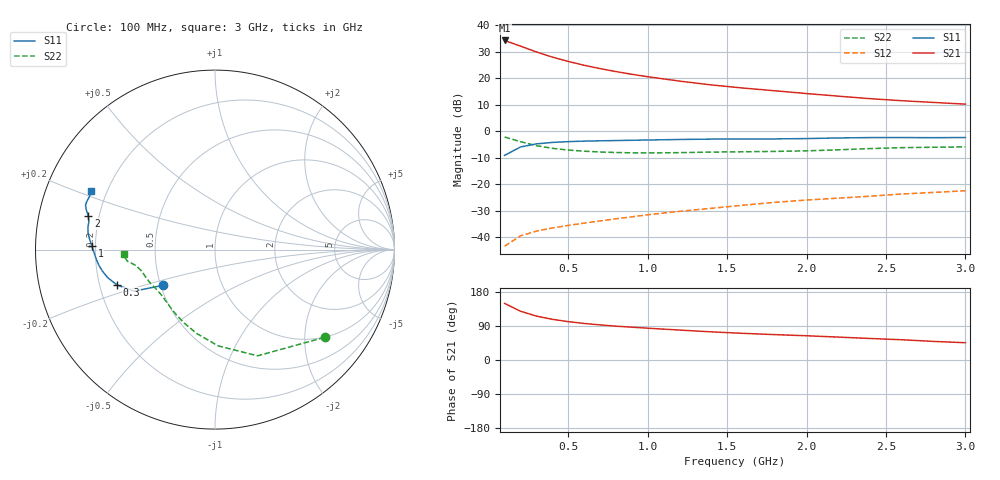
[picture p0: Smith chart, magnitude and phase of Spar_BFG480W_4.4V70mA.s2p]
! Filename: 4_470BFG480.001
! Title: BFG480W
! Bias: Vce=4.4V; Ic=70mA
! Company: NXP Semiconductors NL
! User: Quality&Reliability T&D
! Measure time: 10 Nov 1999 / 12:06:25
#  MHz  S  MA  R 50
! Freq  S11  S21  S12  S22  :
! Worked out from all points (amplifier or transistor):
!   20 points, 100 MHz to 3 GHz, reference 50 ohm
!   highest |S21| = 34.3 dB at 100 MHz (marker M1)
!   |S21| within 3 dB of that: start of sweep to 239.3 MHz
!   unconditionally stable (mu >= 1): 843.2 MHz to end of sweep
!   at 400 MHz: K = 0.73, MSG = 32.3 dB, |S12| = -36.5 dB
!   at 1.2 GHz: K = 1.06, MAG = 23.1 dB, |S12| = -30.2 dB
!   at 3 GHz: K = 1.05, MAG = 15.0 dB, |S12| = -22.4 dB
!   S11 on the Smith chart (normalised r, x): 100 MHz: 0.51, -0.23; 300 MHz: 0.27, -0.16; 1 GHz: 0.19, +0.01; 2 GHz: 0.16, +0.13; 3 GHz: 0.14, +0.22
100  0.3516 -145.5  51.9 149.4  0.006803 67.2  0.782 -38.7
200  0.5065 -152.8  40.58 128.7  0.01065 58.1  0.6376 -68.2
300  0.58 -160.1  31.51 115.9  0.01307 56.0  0.5365 -88.2
400  0.6175 -165.3  25.23 107.4  0.01499 56.5  0.478 -102.4
500  0.6394 -169.3  20.87 101.2  0.01674 58.5  0.4434 -112.9
600  0.6532 -172.4  17.67 96.5  0.01849 60.2  0.4222 -120.8
700  0.6625 -175.1  15.3 92.6  0.02036 62.5  0.4079 -127.0
800  0.6702 -177.4  13.43 89.4  0.02235 64.5  0.3984 -132.2
900  0.6779 -179.6  11.94 86.6  0.02432 66.5  0.393 -136.7
1000  0.6862 178.4  10.74 83.9  0.0266 67.9  0.3912 -140.7
1200  0.7017 175.1  8.878 79.0  0.03086 70.0  0.3962 -147.4
1400  0.7133 172.6  7.522 74.3  0.03525 71.5  0.4055 -152.3
1600  0.7189 170.2  6.562 70.4  0.04028 72.8  0.4113 -156.0
1800  0.7196 167.5  5.835 67.0  0.04574 73.7  0.418 -159.9
2000  0.7302 165.1  5.165 64.0  0.05048 74.7  0.4285 -164.4
2200  0.75 162.9  4.611 60.4  0.05482 74.8  0.4478 -168.3
2400  0.7623 161.1  4.137 56.8  0.05961 74.4  0.4725 -170.9
2600  0.7633 159.5  3.783 53.4  0.06564 74.0  0.4918 -172.4
2800  0.7593 157.2  3.511 49.0  0.07033 72.8  0.501 -174.3
3000  0.7643 154.5  3.26 45.6  0.07564 72.1  0.5085 -177.3
